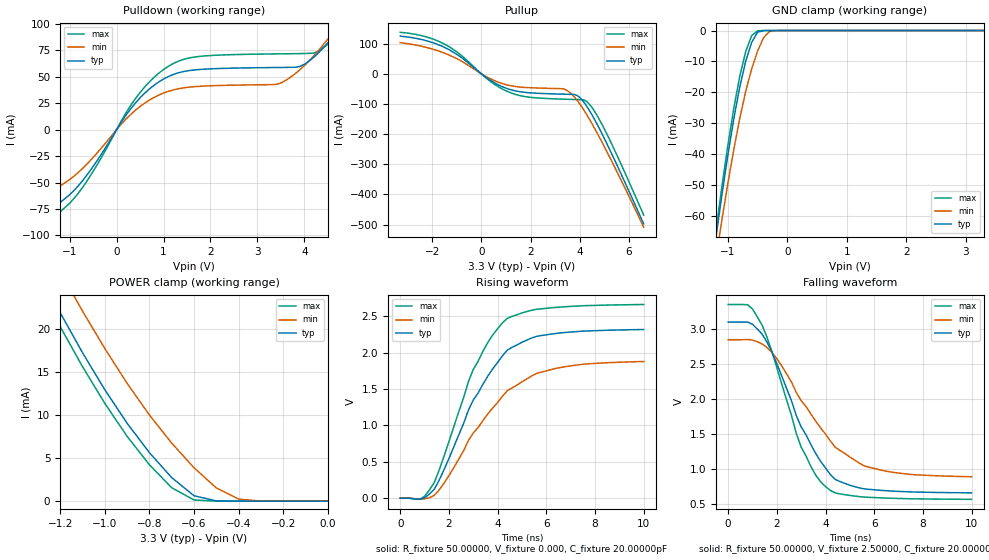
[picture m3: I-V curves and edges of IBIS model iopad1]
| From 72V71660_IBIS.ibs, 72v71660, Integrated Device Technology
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|   Model iopad1
[Model]   iopad1
Model_type   3-state
Polarity   Non-Inverting
Enable   Active-High
|Vinl =  0.80000V
|Vinh =  2.00000V
Vmeas =  1.50000V
C_comp   5.00000pF   NA   NA
[Temperature Range]   25.00000   100.00000   0.000
[Voltage Range]   3.30000V   3.00000V   3.60000V
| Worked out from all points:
|   slope of the pulldown table from 0 to 0.495 V, typ, clamps not added: 16.6 ohm
|   slope of the pullup table from 0 to 0.495 V, typ, clamps not added: 17.8 ohm
|   GND clamp passes 1 mA (typ) near -0.51 V on its own axis
|   POWER clamp passes 1 mA (typ) near -0.62 V on its own axis
|   rising waveform, R_fixture 50.00000, V_fixture 0.000, C_fixture 20.00000pF: 20-80 % time 2.08ns typ, 2.41ns min, 1.83ns max; typ from 0 V to 2.32 V
|   falling waveform, R_fixture 50.00000, V_fixture 2.50000, C_fixture 20.00000pF: 20-80 % time 1.86ns typ, 2.29ns min, 1.6ns max; typ from 3.1 V to 0.664 V
[Pulldown]
| voltage   I(typ)   I(min)   I(max)
-3.3V     -98.4mA    -81.6mA    -110.5mA
-1.9V     -86.7mA    -69mA      -97.4mA
-1.3V     -72.39mA   -56.23mA   -81.63mA
-700mV    -46.93mA   -35.66mA   -53.13mA
500mV     30.12mA    21.95mA    35.15mA
1.3V      53.65mA    38.65mA    64.55mA
3.5V      58.91mA    44.27mA    71.8mA
4V        61.97mA    60.76mA    72.13mA
4.3V      72.71mA    74.98mA    74.18mA
4.7V      93.7mA     97.87mA    90.09mA
4.9V      106.9mA    111.1mA    101.7mA
6.6V      332.3mA    305.7mA    332.7mA
[Pullup]
| voltage   I(typ)   I(min)   I(max)
-3.3V     125.2mA    103.6mA    137.8mA
-2.3V     111.4mA    89.05mA    124mA
-1.5V     87.93mA    68.71mA    98.74mA
400mV     -23.23mA   -17.72mA   -26.94mA
1.2V      -52.73mA   -39.41mA   -63mA
3.3V      -67.33mA   -49.39mA   -83.89mA
3.6V      -67.91mA   -61.92mA   -84.61mA
4V        -78.45mA   -99.51mA   -85.44mA
4.2V      -97.4mA    -124.1mA   -87.42mA
4.5V      -136.2mA   -165.3mA   -111.4mA
5.3V      -265.2mA   -289.4mA   -232.6mA
6.6V      -497.9mA   -508.6mA   -468.4mA
[GND_clamp]
| voltage   I(typ)   I(min)   I(max)
-3.3V     -424.5mA   -403.9mA   -432.6mA
-1.2V     -66.92mA   -73.75mA   -64.72mA
-1.1V     -53.15mA   -61.24mA   -50.45mA
-900mV    -28.53mA   -38.43mA   -25.1mA
-800mV    -18.24mA   -28.42mA   -14.76mA
-700mV    -9.879mA   -19.65mA   -6.761mA
-600mV    -3.823mA   -12.36mA   -1.619mA
-500mV    -522.3uA   -6.579mA   -69.89uA
-400mV    -15.84uA   -2.286mA   -1.491uA
-300mV    -368.6nA   -278.7uA   -29.25nA
-200mV    -8.239nA   -14.25uA   -516.1pA
3.3V      29.26pA    12.72uA    2.135pA
[POWER_clamp]
| voltage   I(typ)   I(min)   I(max)
-3.3V     169.2mA    163.5mA    171.9mA
-1.3V     26.89mA    31.6mA     25.32mA
-1.2V     21.93mA    26.74mA    20.31mA
-1.1V     17.28mA    22.12mA    15.66mA
-1V       12.97mA    17.76mA    11.38mA
-900mV    9.066mA    13.71mA    7.542mA
-800mV    5.637mA    10.02mA    4.237mA
-700mV    2.735mA    6.75mA     1.558mA
-600mV    627uA      3.884mA    134.9uA
-500mV    26.21uA    1.53mA     2.445uA
-400mV    585.2nA    230uA      43.52nA
0V        29.28pA    88.51nA    2.883pA
[Ramp]
| variable   typ   min   max
dV/dt_r   1.39320/1.55145n   1.13040/1.90274n   1.59900/1.32996n
dV/dt_f   1.40130/1.59333n   1.10340/2.00863n   1.61178/1.36973n
R_load = 50.00000
[Rising Waveform]
R_fixture = 50.00000
V_fixture = 0.000
C_fixture = 20.00000pF
R_dut = 129.80000m
L_dut = 9.76000nH
C_dut = 1.23400pF
| time   V(typ)   V(min)   V(max)
0s        0V         0V         0V
800ps     -15.33mV   -14.76mV   -14.41mV
1.4ns     123.7mV    40.45mV    217mV
2ns       545.2mV    310.4mV    777mV
3ns       1.348V     895.9mV    1.767V
3.8ns     1.776V     1.239V     2.242V
4.4ns     2.034V     1.476V     2.47V
5.6ns     2.223V     1.714V     2.595V
6.4ns     2.263V     1.782V     2.62V
10ns      2.316V     1.877V     2.66V
[Falling Waveform]
R_fixture = 50.00000
V_fixture = 2.50000
C_fixture = 20.00000pF
R_dut = 129.80000m
L_dut = 9.76000nH
C_dut = 1.23400pF
| time   V(typ)   V(min)   V(max)
0s        3.103V     2.852V     3.355V
800ps     3.105V     2.855V     3.352V
1.4ns     2.929V     2.791V     3.056V
2ns       2.51V      2.582V     2.454V
3ns       1.606V     1.981V     1.316V
3.6ns     1.225V     1.687V     915.6mV
4ns       1.019V     1.503V     753mV
4.4ns     855.4mV    1.315V     662.5mV
5.6ns     719.8mV    1.048V     602.8mV
10ns      663.6mV    894.1mV    571mV
